(* Logix 5000 DataType export ZE2AI_Seneca_InData; software revision 35.00 *)

TYPE ZE2AI_Seneca_InData :   // User Define Measure Data Type for Seneca ZE-2AI-E Device
STRUCT
   AIN1 : REAL;
   AIN2 : REAL;
   FLAGS : INT;
END_STRUCT
END_TYPE
